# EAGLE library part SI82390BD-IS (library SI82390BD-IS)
Gate Drivers 5 kV 8 V UVLO dual isolated gate driver Source: Datasheet
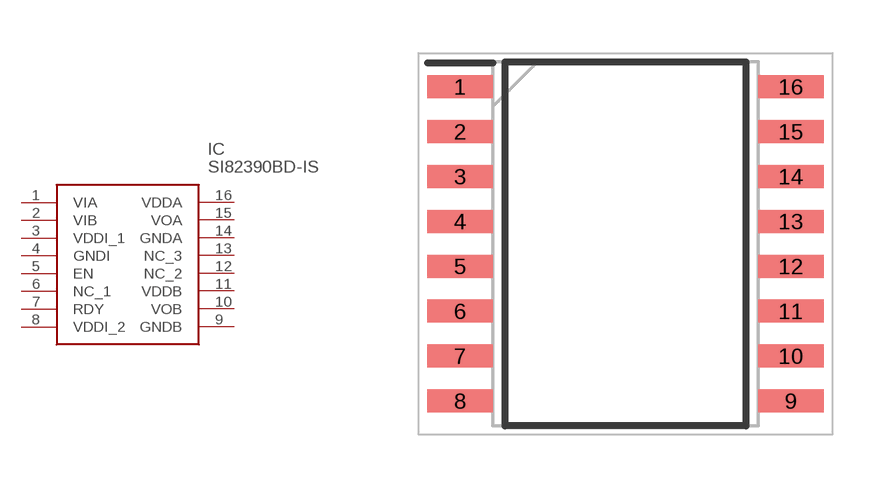
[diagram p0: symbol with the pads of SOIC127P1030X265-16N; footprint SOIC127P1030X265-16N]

Designator prefix IC

## SI82390BD-IS (Description: Gate Drivers 5 kV 8 V UVLO dual isolated gate driver; Height: 2.65mm; Manufacturer_Name: Skyworks; Manufacturer_Part_Number: SI82390BD-IS; Mouser_Part_Number: 634-SI82390BD-IS; Mouser_Price-Stock: https://www.mouser.co.uk/ProductDetail/Skyworks-Solutions-Inc/SI82390BD-IS?qs=6OIXIgk3fwek%2FlEM9Z8%2F2g%3D%3D)  [SOIC127P1030X265-16N]
1  VIA
2  VIB
3  VDDI_1
4  GNDI
5  EN
6  NC_1
7  RDY
8  VDDI_2
9  GNDB
10  VOB
11  VDDB
12  NC_2
13  NC_3
14  GNDA
15  VOA
16  VDDA

## Footprint SOIC127P1030X265-16N (pad centres in mm)
16-Pin Wide Body SOIC_2021
smd 1.85 x 0.65: 1 -4.675,4.445; 2 -4.675,3.175; 3 -4.675,1.905; 4 -4.675,0.635; 5 -4.675,-0.635; 6 -4.675,-1.905; 7 -4.675,-3.175; 8 -4.675,-4.445; 9 4.675,-4.445; 10 4.675,-3.175; 11 4.675,-1.905; 12 4.675,-0.635; 13 4.675,0.635; 14 4.675,1.905; 15 4.675,3.175; 16 4.675,4.445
